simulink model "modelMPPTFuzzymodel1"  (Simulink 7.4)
settings: Solver=ode1  SolverMode=SingleTasking  StartTime=0.0  StopTime=10  FixedStep=1e-4  MaxStep=1e-5
libraries: fuzblock x1

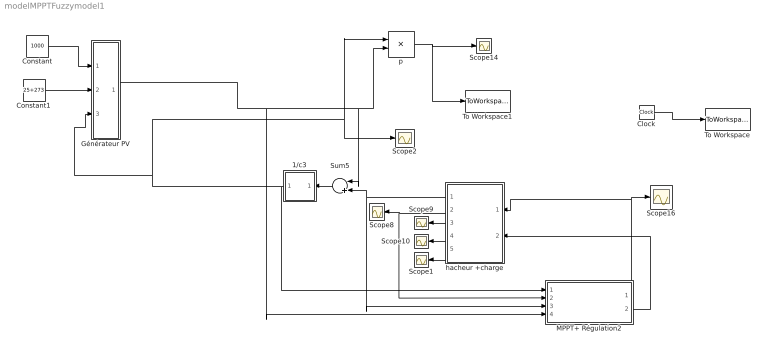
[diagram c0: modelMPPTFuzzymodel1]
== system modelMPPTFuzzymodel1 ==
  1/c3 : Subsystem
  Clock : Clock
  Constant : Constant  Value=1000  OutDataType=sfix(16)  OutScaling=2^0
  Constant1 : Constant  Value=25+273  OutDataType=sfix(16)  OutScaling=2^0
  Générateur PV : Subsystem
  MPPT+ Régulation2 : Subsystem
  Scope{1..2,8..10,14,16} (7 alike) : Scope
  Sum5 : Sum  Inputs=|+-  OutDataType=sfix(16)  OutScaling=2^0
  To Workspace : ToWorkspace  VariableName=t  SampleTime=-1  SaveFormat=Array
  To Workspace1 : ToWorkspace  VariableName=P  SampleTime=-1  SaveFormat=Array
  hacheur +charge : Subsystem
  p : Product  OutDataType=sfix(16)  OutScaling=2^0
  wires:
  1/c3/1(Vdc) -> MPPT+ Régulation2/1(vpv), Générateur PV/3(VG), p/1, Scope2/1
  hacheur +charge/3(iCH) -> Scope9/1
  hacheur +charge/4(Pch) -> Scope10/1
  hacheur +charge/2(Vch) -> Scope8/1, MPPT+ Régulation2/2(vch)
  MPPT+ Régulation2/1(1-alpha) -> hacheur +charge/1(" 1-alpha"), Scope16/1
  MPPT+ Régulation2/2(VPV1) -> hacheur +charge/2(vpv)
  p/1 -> Scope14/1, To Workspace1/1
  hacheur +charge/5(iL'1) -> Scope1/1
  hacheur +charge/1(iL) -> Sum5/2, MPPT+ Régulation2/3(il)
  Clock/1 -> To Workspace/1
  Sum5/1 -> 1/c3/1(Idc)
  Générateur PV/1(IG) -> MPPT+ Régulation2/4(ipv), p/2, Sum5/1
  Constant/1 -> Générateur PV/1(Es)
  Constant1/1 -> Générateur PV/2(Tj)

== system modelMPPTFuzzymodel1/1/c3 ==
  Idc : Inport  OutDataType=sfix(16)  OutScaling=2^0
  Gain : Gain  Gain=1/900e-5  ParameterDataType=sfix(16)  ParameterScaling=2^0  OutDataType=sfix(16)  OutScaling=2^0
  Integrator : Integrator
  Vdc : Outport
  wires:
  Gain/1 -> Integrator/1
  Idc/1 -> Gain/1
  Integrator/1 -> Vdc/1

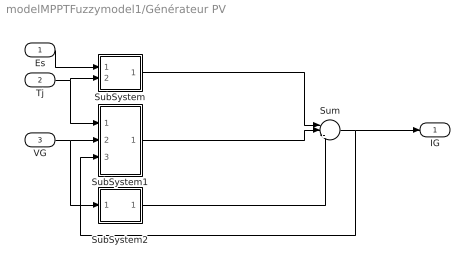
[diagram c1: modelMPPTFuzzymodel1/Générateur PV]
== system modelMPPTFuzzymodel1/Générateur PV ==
  Es : Inport  OutDataType=sfix(16)  OutScaling=2^0
  Tj : Inport  Port=2  OutDataType=sfix(16)  OutScaling=2^0
  VG : Inport  Port=3  OutDataType=sfix(16)  OutScaling=2^0
  SubSystem : Subsystem  mask{Tjref=298, Eref=1000, p3=-0.336e-4, p2=0.58e-5, p1=0.00345}
      mask prompts: Tjref "Tjref[°k]"; Eref "Eref[W/m^2]"
  SubSystem1 : Subsystem  mask{Rs=0.92251, ns=72, p4=31.2367, Eg=1.76e-19, q=1.6e-19, A=1, k=1.38e-23}
      mask prompts: Rs "Rs[ohm]"; q "q[C]"; k "k[J/°K]"
  SubSystem2 : Subsystem  mask{Rsh=235.1551}
      mask prompts: Rsh "Rsh[ohm]"
  Sum : Sum  Inputs=|+--  OutDataType=sfix(16)  OutScaling=2^0
  IG : Outport  OutDataType=sfix(16)  OutScaling=2^0
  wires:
  SubSystem/1(Iph) -> Sum/1
  SubSystem1/1(Id) -> Sum/2
  SubSystem2/1(Irsh) -> Sum/3
  Es/1 -> SubSystem/1(Es)
  Tj/1 -> SubSystem/2(Tj), SubSystem1/1(Tj)
  Sum/1 -> IG/1, SubSystem1/3(IG)
  VG/1 -> SubSystem1/2(VG), SubSystem2/1(VG)

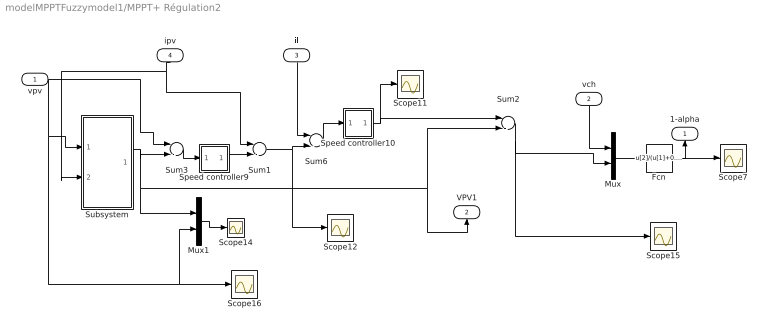
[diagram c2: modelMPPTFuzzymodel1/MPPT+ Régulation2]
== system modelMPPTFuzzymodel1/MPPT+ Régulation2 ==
  vpv : Inport  OutDataType=sfix(16)  OutScaling=2^0
  vch : Inport  Port=2  OutDataType=sfix(16)  OutScaling=2^0
  il : Inport  Port=3  OutDataType=sfix(16)  OutScaling=2^0
  ipv : Inport  Port=4  OutDataType=sfix(16)  OutScaling=2^0
  Fcn : Fcn  Expr=u[2]/(u[1]+0.1)
  Mux : Mux  Inputs=2
  Mux1 : Mux  Inputs=2
  Scope{7,11..12,14..16} (6 alike) : Scope
  Speed controller10 : Subsystem  mask{Kp2=0.01, Ki2=0.1963}
      mask prompts: Kp2 "Proportional gain (Kp)"; Ki2 "Integral gain (Ki)"
      mask help: Proportional-Integral Speed Controller
  Speed controller9 : Subsystem  mask{Kp2=7, Ki2=33.62}
      mask prompts: Kp2 "Proportional gain (Kp)"; Ki2 "Integral gain (Ki)"
      mask help: Proportional-Integral Speed Controller
  Subsystem : Subsystem
  Sum{1..3,6} (4 alike) : Sum  Inputs=|-+  OutDataType=sfix(16)  OutScaling=2^0
  1-alpha : Outport
  VPV1 : Outport  Port=2
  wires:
  Mux1/1 -> Scope14/1
  Subsystem/1(Vref) -> Mux1/1, VPV1/1, Sum2/2, Sum3/2
  Speed controller9/1(Ura) -> Sum1/2
  vpv/1 -> Sum3/1, Scope16/1, Mux1/2, Subsystem/1(Vpv)
  Sum1/1 -> Scope12/1, Sum6/2
  vch/1 -> Mux/1
  Sum2/1 -> Mux/2, Scope15/1
  Fcn/1 -> 1-alpha/1, Scope7/1
  Mux/1 -> Fcn/1
  Speed controller10/1(Ura) -> Sum2/1, Scope11/1
  Sum6/1 -> Speed controller10/1(Ia)
  ipv/1 -> Sum1/1, Subsystem/2(Ipv)
  Sum3/1 -> Speed controller9/1(Ia)
  il/1 -> Sum6/1

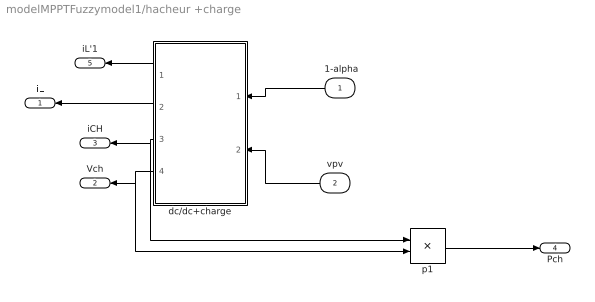
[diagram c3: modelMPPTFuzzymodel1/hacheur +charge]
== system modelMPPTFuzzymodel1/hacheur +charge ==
  " 1-alpha" : Inport  OutDataType=sfix(16)  OutScaling=2^0
  vpv : Inport  Port=2  OutDataType=sfix(16)  OutScaling=2^0
  dc/dc+charge : Subsystem
  p1 : Product  OutDataType=sfix(16)  OutScaling=2^0
  iL : Outport
  Vch : Outport  Port=2
  iCH : Outport  Port=3
  Pch : Outport  Port=4
  iL'1 : Outport  Port=5
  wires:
  vpv/1 -> dc/dc+charge/2(vcpv)
  dc/dc+charge/3(iCH) -> iCH/1, p1/1
  dc/dc+charge/4(Vch) -> Vch/1, p1/2
  p1/1 -> Pch/1
  dc/dc+charge/2(iL) -> iL/1
  " 1-alpha"/1 -> dc/dc+charge/1(1-alpha)
  dc/dc+charge/1(iL'1) -> iL'1/1

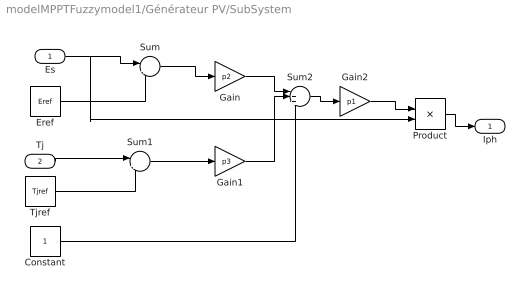
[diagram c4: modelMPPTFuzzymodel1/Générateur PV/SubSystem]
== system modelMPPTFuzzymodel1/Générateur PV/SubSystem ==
  Es : Inport  OutDataType=sfix(16)  OutScaling=2^0
  Tj : Inport  Port=2  OutDataType=sfix(16)  OutScaling=2^0
  Constant : Constant  OutDataType=sfix(16)  OutScaling=2^0
  Eref : Constant  Value=Eref  OutDataType=sfix(16)  OutScaling=2^0
  Gain : Gain  Gain=p2  ParameterDataType=sfix(16)  ParameterScaling=2^0  OutDataType=sfix(16)  OutScaling=2^0
  Gain1 : Gain  Gain=p3  ParameterDataType=sfix(16)  ParameterScaling=2^0  OutDataType=sfix(16)  OutScaling=2^0
  Gain2 : Gain  Gain=p1  ParameterDataType=sfix(16)  ParameterScaling=2^0  OutDataType=sfix(16)  OutScaling=2^0
  Product : Product  OutDataType=sfix(16)  OutScaling=2^0
  Sum : Sum  Inputs=|+-  OutDataType=sfix(16)  OutScaling=2^0
  Sum1 : Sum  Inputs=|+-  OutDataType=sfix(16)  OutScaling=2^0
  Sum2 : Sum  Inputs=|+++  OutDataType=sfix(16)  OutScaling=2^0
  Tjref : Constant  Value=Tjref  OutDataType=sfix(16)  OutScaling=2^0
  Iph : Outport  OutDataType=sfix(16)  OutScaling=2^0
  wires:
  Eref/1 -> Sum/2
  Tj/1 -> Sum1/1
  Tjref/1 -> Sum1/2
  Sum/1 -> Gain/1
  Sum1/1 -> Gain1/1
  Gain/1 -> Sum2/1
  Gain1/1 -> Sum2/2
  Constant/1 -> Sum2/3
  Sum2/1 -> Gain2/1
  Gain2/1 -> Product/1
  Es/1 -> Sum/1, Product/2
  Product/1 -> Iph/1

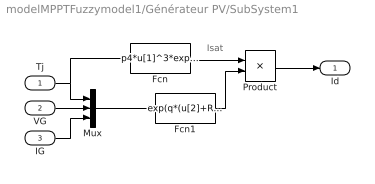
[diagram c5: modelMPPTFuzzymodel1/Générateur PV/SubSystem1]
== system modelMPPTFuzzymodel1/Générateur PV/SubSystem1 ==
  note: Isat
  Tj : Inport  OutDataType=sfix(16)  OutScaling=2^0
  VG : Inport  Port=2  OutDataType=sfix(16)  OutScaling=2^0
  IG : Inport  Port=3  OutDataType=sfix(16)  OutScaling=2^0
  Fcn : Fcn  Expr=p4*u[1]^3*exp(-Eg/(k*u[1]))
  Fcn1 : Fcn  Expr=exp(q*(u[2]+Rs*u[3])/(k*A*ns*u[1]))-1
  Mux : Mux  Inputs=3
  Product : Product  OutDataType=sfix(16)  OutScaling=2^0
  Id : Outport  OutDataType=sfix(16)  OutScaling=2^0
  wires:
  Mux/1 -> Fcn1/1
  Fcn/1 -> Product/1
  Fcn1/1 -> Product/2
  Product/1 -> Id/1
  VG/1 -> Mux/2
  IG/1 -> Mux/3
  Tj/1 -> Mux/1, Fcn/1

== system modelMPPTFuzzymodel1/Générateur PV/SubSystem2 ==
  VG : Inport  OutDataType=sfix(16)  OutScaling=2^0
  Gain : Gain  Gain=1/Rsh  ParameterDataType=sfix(16)  ParameterScaling=2^0  OutDataType=sfix(16)  OutScaling=2^0
  Irsh : Outport  OutDataType=sfix(16)  OutScaling=2^0
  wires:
  VG/1 -> Gain/1
  Gain/1 -> Irsh/1

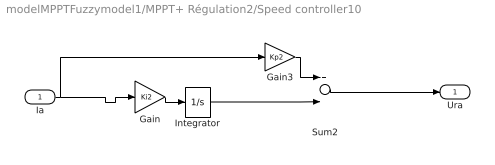
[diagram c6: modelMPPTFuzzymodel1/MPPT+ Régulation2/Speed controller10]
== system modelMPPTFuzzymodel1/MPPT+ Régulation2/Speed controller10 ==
  Ia : Inport  OutDataType=sfix(16)  OutScaling=2^0
  Gain : Gain  Gain=Ki2  ParameterDataType=sfix(16)  ParameterScaling=2^0  OutDataType=sfix(16)  OutScaling=2^0
  Gain3 : Gain  Gain=Kp2  ParameterDataType=sfix(16)  ParameterScaling=2^0  OutDataType=sfix(16)  OutScaling=2^0
  Integrator : Integrator  UpperSaturationLimit=30  LowerSaturationLimit=-30
  Sum2 : Sum  OutDataType=sfix(16)  OutScaling=2^0
  Ura : Outport  InitialOutput=0
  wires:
  Gain/1 -> Integrator/1
  Gain3/1 -> Sum2/1
  Sum2/1 -> Ura/1
  Integrator/1 -> Sum2/2
  Ia/1 -> Gain/1, Gain3/1

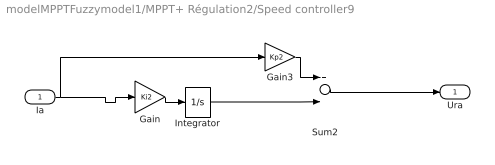
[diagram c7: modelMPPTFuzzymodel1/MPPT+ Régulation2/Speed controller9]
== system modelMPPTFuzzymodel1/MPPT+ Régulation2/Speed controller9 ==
  Ia : Inport  OutDataType=sfix(16)  OutScaling=2^0
  Gain : Gain  Gain=Ki2  ParameterDataType=sfix(16)  ParameterScaling=2^0  OutDataType=sfix(16)  OutScaling=2^0
  Gain3 : Gain  Gain=Kp2  ParameterDataType=sfix(16)  ParameterScaling=2^0  OutDataType=sfix(16)  OutScaling=2^0
  Integrator : Integrator  UpperSaturationLimit=30  LowerSaturationLimit=-30
  Sum2 : Sum  OutDataType=sfix(16)  OutScaling=2^0
  Ura : Outport  InitialOutput=0
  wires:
  Ia/1 -> Gain3/1, Gain/1
  Integrator/1 -> Sum2/2
  Sum2/1 -> Ura/1
  Gain3/1 -> Sum2/1
  Gain/1 -> Integrator/1

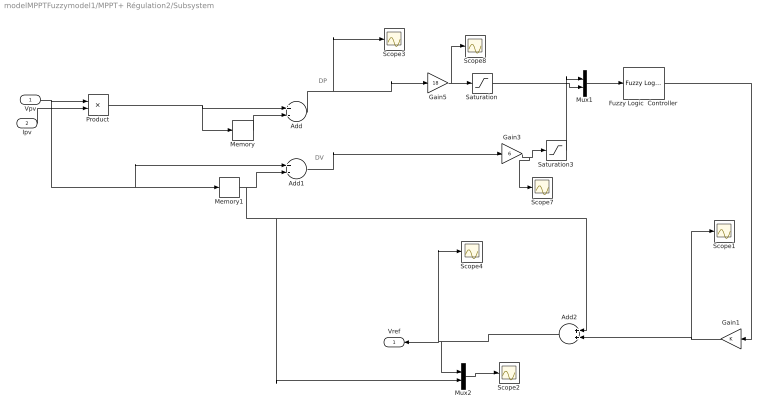
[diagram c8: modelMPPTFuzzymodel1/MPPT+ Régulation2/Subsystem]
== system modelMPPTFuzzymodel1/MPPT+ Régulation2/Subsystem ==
  note: DP
  note: DV
  Vpv : Inport
  Ipv : Inport  Port=2
  Add : Sum  Inputs=+-  OutDataType=sfix(16)  OutScaling=2^-10
  Add1 : Sum  Inputs=+-  OutDataType=sfix(16)  OutScaling=2^-10
  Add2 : Sum  OutDataType=sfix(16)  OutScaling=2^-10
  Fuzzy Logic  Controller : fuzblock/Fuzzy Logic  Controller  SystemSampleTime=-1  fis=SAMM
  Gain1 : Gain  ParameterDataType=sfix(16)  ParameterScaling=2^0  OutDataType=sfix(16)  OutScaling=2^0
  Gain3 : Gain  Gain=6  ParameterDataType=sfix(16)  ParameterScaling=2^0  OutDataType=sfix(16)  OutScaling=2^0
  Gain5 : Gain  Gain=18  ParameterDataType=sfix(16)  ParameterScaling=2^0  OutDataType=sfix(16)  OutScaling=2^0
  Memory : Memory
  Memory1 : Memory
  Mux1 : Mux  Inputs=2
  Mux2 : Mux  Inputs=2
  Product : Product  OutDataType=sfix(16)  OutScaling=2^0
  Saturation : Saturate  UpperLimit=1  LowerLimit=-1  OutDataType=sfix(16)  OutScaling=2^0
  Saturation3 : Saturate  UpperLimit=1  LowerLimit=-1  OutDataType=sfix(16)  OutScaling=2^0
  Scope{1..4,7..8} (6 alike) : Scope
  Vref : Outport  OutDataType=sfix(16)  OutScaling=2^0
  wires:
  Memory/1 -> Add/2
  Memory1/1 -> Add1/2, Add2/1, Mux2/2
  Fuzzy Logic  Controller/1 -> Gain1/1
  Add1/1 -> Gain3/1
  Product/1 -> Add/1, Memory/1
  Add/1 -> Scope3/1, Gain5/1
  Gain5/1 -> Scope8/1, Saturation/1
  Mux1/1 -> Fuzzy Logic  Controller/1
  Gain3/1 -> Scope7/1, Saturation3/1
  Gain1/1 -> Scope1/1, Add2/2
  Vpv/1 -> Memory1/1, Add1/1, Product/1
  Ipv/1 -> Product/2
  Saturation3/1 -> Mux1/1
  Saturation/1 -> Mux1/2
  Add2/1 -> Vref/1, Scope4/1, Mux2/1
  Mux2/1 -> Scope2/1

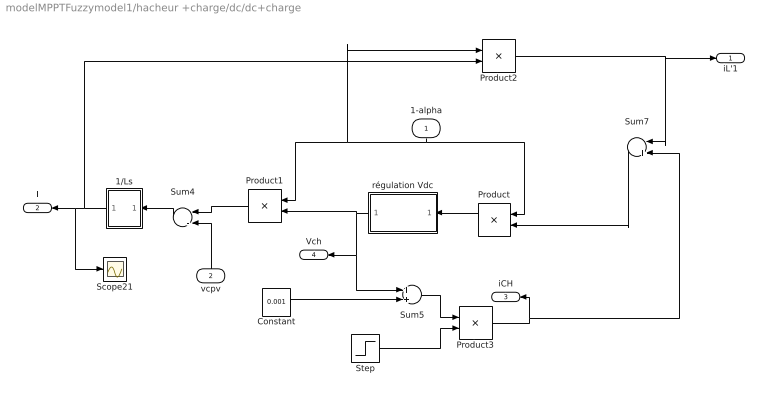
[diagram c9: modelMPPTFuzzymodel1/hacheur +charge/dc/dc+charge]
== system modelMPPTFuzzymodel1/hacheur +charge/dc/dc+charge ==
  1-alpha : Inport  OutDataType=sfix(16)  OutScaling=2^0
  vcpv : Inport  Port=2  OutDataType=sfix(16)  OutScaling=2^0
  1/Ls : Subsystem
  Constant : Constant  Value=0.001  OutDataType=sfix(16)  OutScaling=2^0
  Product : Product  OutDataType=sfix(16)  OutScaling=2^0
  Product1 : Product  OutDataType=sfix(16)  OutScaling=2^0
  Product2 : Product  OutDataType=sfix(16)  OutScaling=2^0
  Product3 : Product  Inputs=/*  OutDataType=sfix(16)  OutScaling=2^0
  Scope21 : Scope
  Step : Step  Before=70  After=70  SampleTime=0
  Sum4 : Sum  Inputs=|-+  OutDataType=sfix(16)  OutScaling=2^0
  Sum5 : Sum  OutDataType=sfix(16)  OutScaling=2^0
  Sum7 : Sum  Inputs=|+-  OutDataType=sfix(16)  OutScaling=2^0
  régulation Vdc : Subsystem
  iL'1 : Outport
  iL : Outport  Port=2
  iCH : Outport  Port=3
  Vch : Outport  Port=4
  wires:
  régulation Vdc/1(Vdc) -> Product1/2, Vch/1, Sum5/1
  Sum7/1 -> Product/2
  1-alpha/1 -> Product/1, Product1/1, Product2/1
  Sum4/1 -> 1/Ls/1(ul)
  vcpv/1 -> Sum4/2
  Product/1 -> régulation Vdc/1(Idc)
  Product1/1 -> Sum4/1
  1/Ls/1(il) -> iL/1, Scope21/1, Product2/2
  Product2/1 -> Sum7/1, iL'1/1
  Step/1 -> Product3/2
  Product3/1 -> iCH/1, Sum7/2
  Sum5/1 -> Product3/1
  Constant/1 -> Sum5/2

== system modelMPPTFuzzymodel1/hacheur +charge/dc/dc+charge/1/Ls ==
  ul : Inport  OutDataType=sfix(16)  OutScaling=2^0
  Gain : Gain  Gain=1/0.66e-5  ParameterDataType=sfix(16)  ParameterScaling=2^0  OutDataType=sfix(16)  OutScaling=2^0
  Integrator : Integrator
  il : Outport
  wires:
  Integrator/1 -> il/1
  ul/1 -> Gain/1
  Gain/1 -> Integrator/1

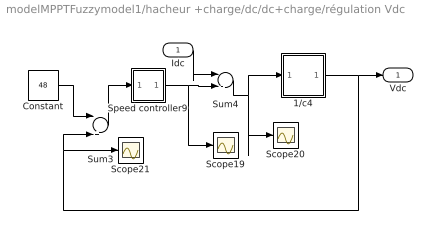
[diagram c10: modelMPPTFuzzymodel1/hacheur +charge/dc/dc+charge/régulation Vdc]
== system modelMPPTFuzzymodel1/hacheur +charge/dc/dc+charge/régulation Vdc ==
  Idc : Inport  OutDataType=sfix(16)  OutScaling=2^0
  1/c4 : Subsystem
  Constant : Constant  Value=48  OutDataType=sfix(16)  OutScaling=2^0
  Scope19 : Scope
  Scope20 : Scope
  Scope21 : Scope
  Speed controller9 : Subsystem  mask{Kp2=98, Ki2=220}
      mask prompts: Kp2 "Proportional gain (Kp)"; Ki2 "Integral gain (Ki)"
      mask help: Proportional-Integral Speed Controller
  Sum3 : Sum  Inputs=|+-  OutDataType=sfix(16)  OutScaling=2^0
  Sum4 : Sum  Inputs=|-+  OutDataType=sfix(16)  OutScaling=2^0
  Vdc : Outport
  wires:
  Sum3/1 -> Speed controller9/1(Ia)
  Constant/1 -> Sum3/1
  Idc/1 -> Sum4/1
  1/c4/1(Vdc) -> Vdc/1, Sum3/2, Scope21/1
  Speed controller9/1(Ura) -> Sum4/2, Scope19/1
  Sum4/1 -> 1/c4/1(Idc), Scope20/1

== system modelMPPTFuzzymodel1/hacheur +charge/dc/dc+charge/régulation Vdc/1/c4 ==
  Idc : Inport  OutDataType=sfix(16)  OutScaling=2^0
  Gain : Gain  Gain=1/900e-5  ParameterDataType=sfix(16)  ParameterScaling=2^0  OutDataType=sfix(16)  OutScaling=2^0
  Integrator : Integrator
  Vdc : Outport
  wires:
  Gain/1 -> Integrator/1
  Idc/1 -> Gain/1
  Integrator/1 -> Vdc/1

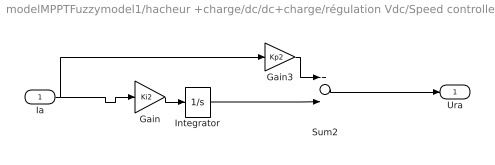
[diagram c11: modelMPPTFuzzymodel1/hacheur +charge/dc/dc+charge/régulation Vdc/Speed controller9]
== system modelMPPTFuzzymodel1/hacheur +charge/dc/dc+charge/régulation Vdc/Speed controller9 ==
  Ia : Inport  OutDataType=sfix(16)  OutScaling=2^0
  Gain : Gain  Gain=Ki2  ParameterDataType=sfix(16)  ParameterScaling=2^0  OutDataType=sfix(16)  OutScaling=2^0
  Gain3 : Gain  Gain=Kp2  ParameterDataType=sfix(16)  ParameterScaling=2^0  OutDataType=sfix(16)  OutScaling=2^0
  Integrator : Integrator  UpperSaturationLimit=30  LowerSaturationLimit=-30
  Sum2 : Sum  OutDataType=sfix(16)  OutScaling=2^0
  Ura : Outport  InitialOutput=0
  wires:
  Ia/1 -> Gain3/1, Gain/1
  Integrator/1 -> Sum2/2
  Sum2/1 -> Ura/1
  Gain3/1 -> Sum2/1
  Gain/1 -> Integrator/1
